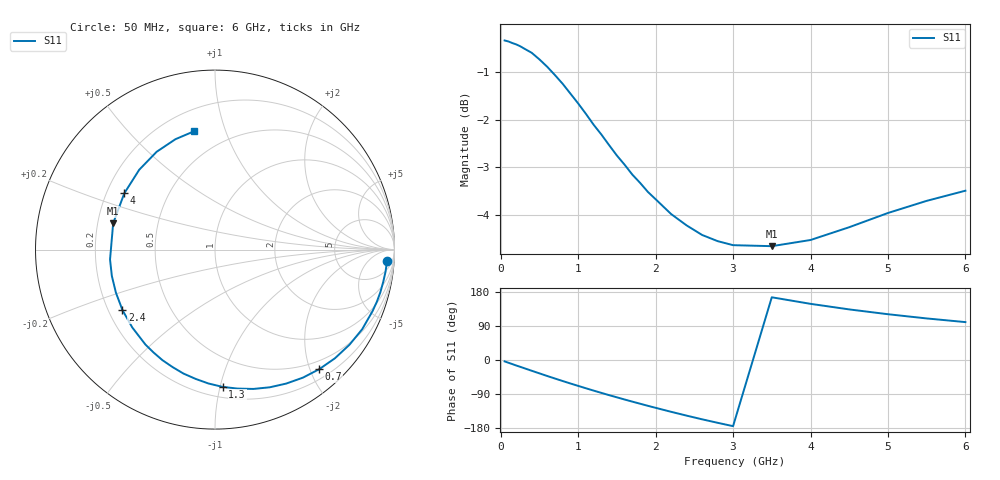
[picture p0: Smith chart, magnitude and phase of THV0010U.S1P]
! SIEMENS Discrete & RF Semiconductors
! BAS70
! Si Schottky Diode in SOT23
! IF = 0.01 mA
! S-Parameters:  February  1997
# GHz  S  MA  R  50
!  f  S11
! GHz  MAG  ANG
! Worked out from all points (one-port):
!   34 points, 50 MHz to 6 GHz, reference 50 ohm
!   lowest |S11| = -4.6 dB at 3.5 GHz (marker M1), VSWR 3.83, Z = 13.2 + j5.92 ohm
!   |S11| at or under -10 dB: nowhere
!   S11 on the Smith chart (normalised r, x): 50 MHz: 14, -22; 700 MHz: 0.35, -2.15; 1.3 GHz: 0.28, -1.02; 2.4 GHz: 0.26, -0.28; 4 GHz: 0.27, +0.27; 6 GHz: 0.33, +0.78
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0.05  0.9605 -3.7
0.15  0.9545 -10.8
0.25  0.9474 -17.9
0.4  0.9324 -28.4
0.5  0.9177 -35.3
0.6  0.9017 -42.2
0.7  0.8838 -48.9
0.8  0.8655 -55.5
0.9  0.8453 -62.0
1  0.8256 -68.3
1.1  0.8052 -74.6
1.2  0.7844 -80.8
1.3  0.7661 -86.8
1.4  0.7469 -92.8
1.6  0.7126 -104.3
1.8  0.6822 -115.4
2  0.6559 -126.2
2.2  0.633 -136.7
2.4  0.616 -146.8
2.6  0.602 -156.5
2.8  0.5932 -165.7
3  0.5874 -174.6
3.5  0.586 165.5
4  0.5948 148.2
4.5  0.6133 133.5
5  0.6346 120.8
5.5  0.6534 109.7
6  0.6695 100.0
